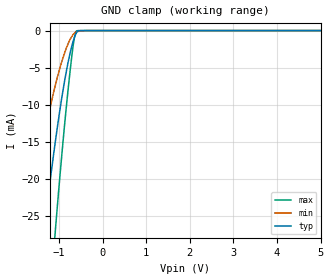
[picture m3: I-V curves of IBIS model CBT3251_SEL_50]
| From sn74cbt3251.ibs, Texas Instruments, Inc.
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[Model]   CBT3251_SEL_50
Model_type  Input
Vinl=0.8
Vinh=2.0
| variable   typ   min   max
C_comp   3.73pF   2.55pF   9.17pF
[Temperature Range]   40   100   -40
| Ambient temperature   25   85   -40
[Voltage range]   5   4.5   5.5
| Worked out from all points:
|   GND clamp passes 1 mA (typ) near -0.65 V on its own axis
[GND Clamp]
| CBT3251_SEL_50
|   Voltage   I(typ)   I(min)   I(max)
-5V       -263mA     -174.2mA   -399.1mA
-1.73V    -47.63mA   -26.98mA   -79.57mA
-1.37V    -28.36mA   -15.13mA   -49.07mA
-1.325V   -26.12mA   -13.8mA    -45.44mA
-1.09V    -15.24mA   -7.519mA   -27.45mA
-1.07V    -14.39mA   -7.046mA   -26mA
-925mV    -8.68mA    -3.968mA   -16.08mA
-765mV    -3.557mA   -1.439mA   -6.511mA
-660mV    -1.157mA   -431.3uA   -1.426mA
-630mV    -669.8uA   -264.7uA   -520.2uA
-595mV    -251.3uA   -151.7uA   -36uA
5V        153.3pA    266.7pA    139.8pA
